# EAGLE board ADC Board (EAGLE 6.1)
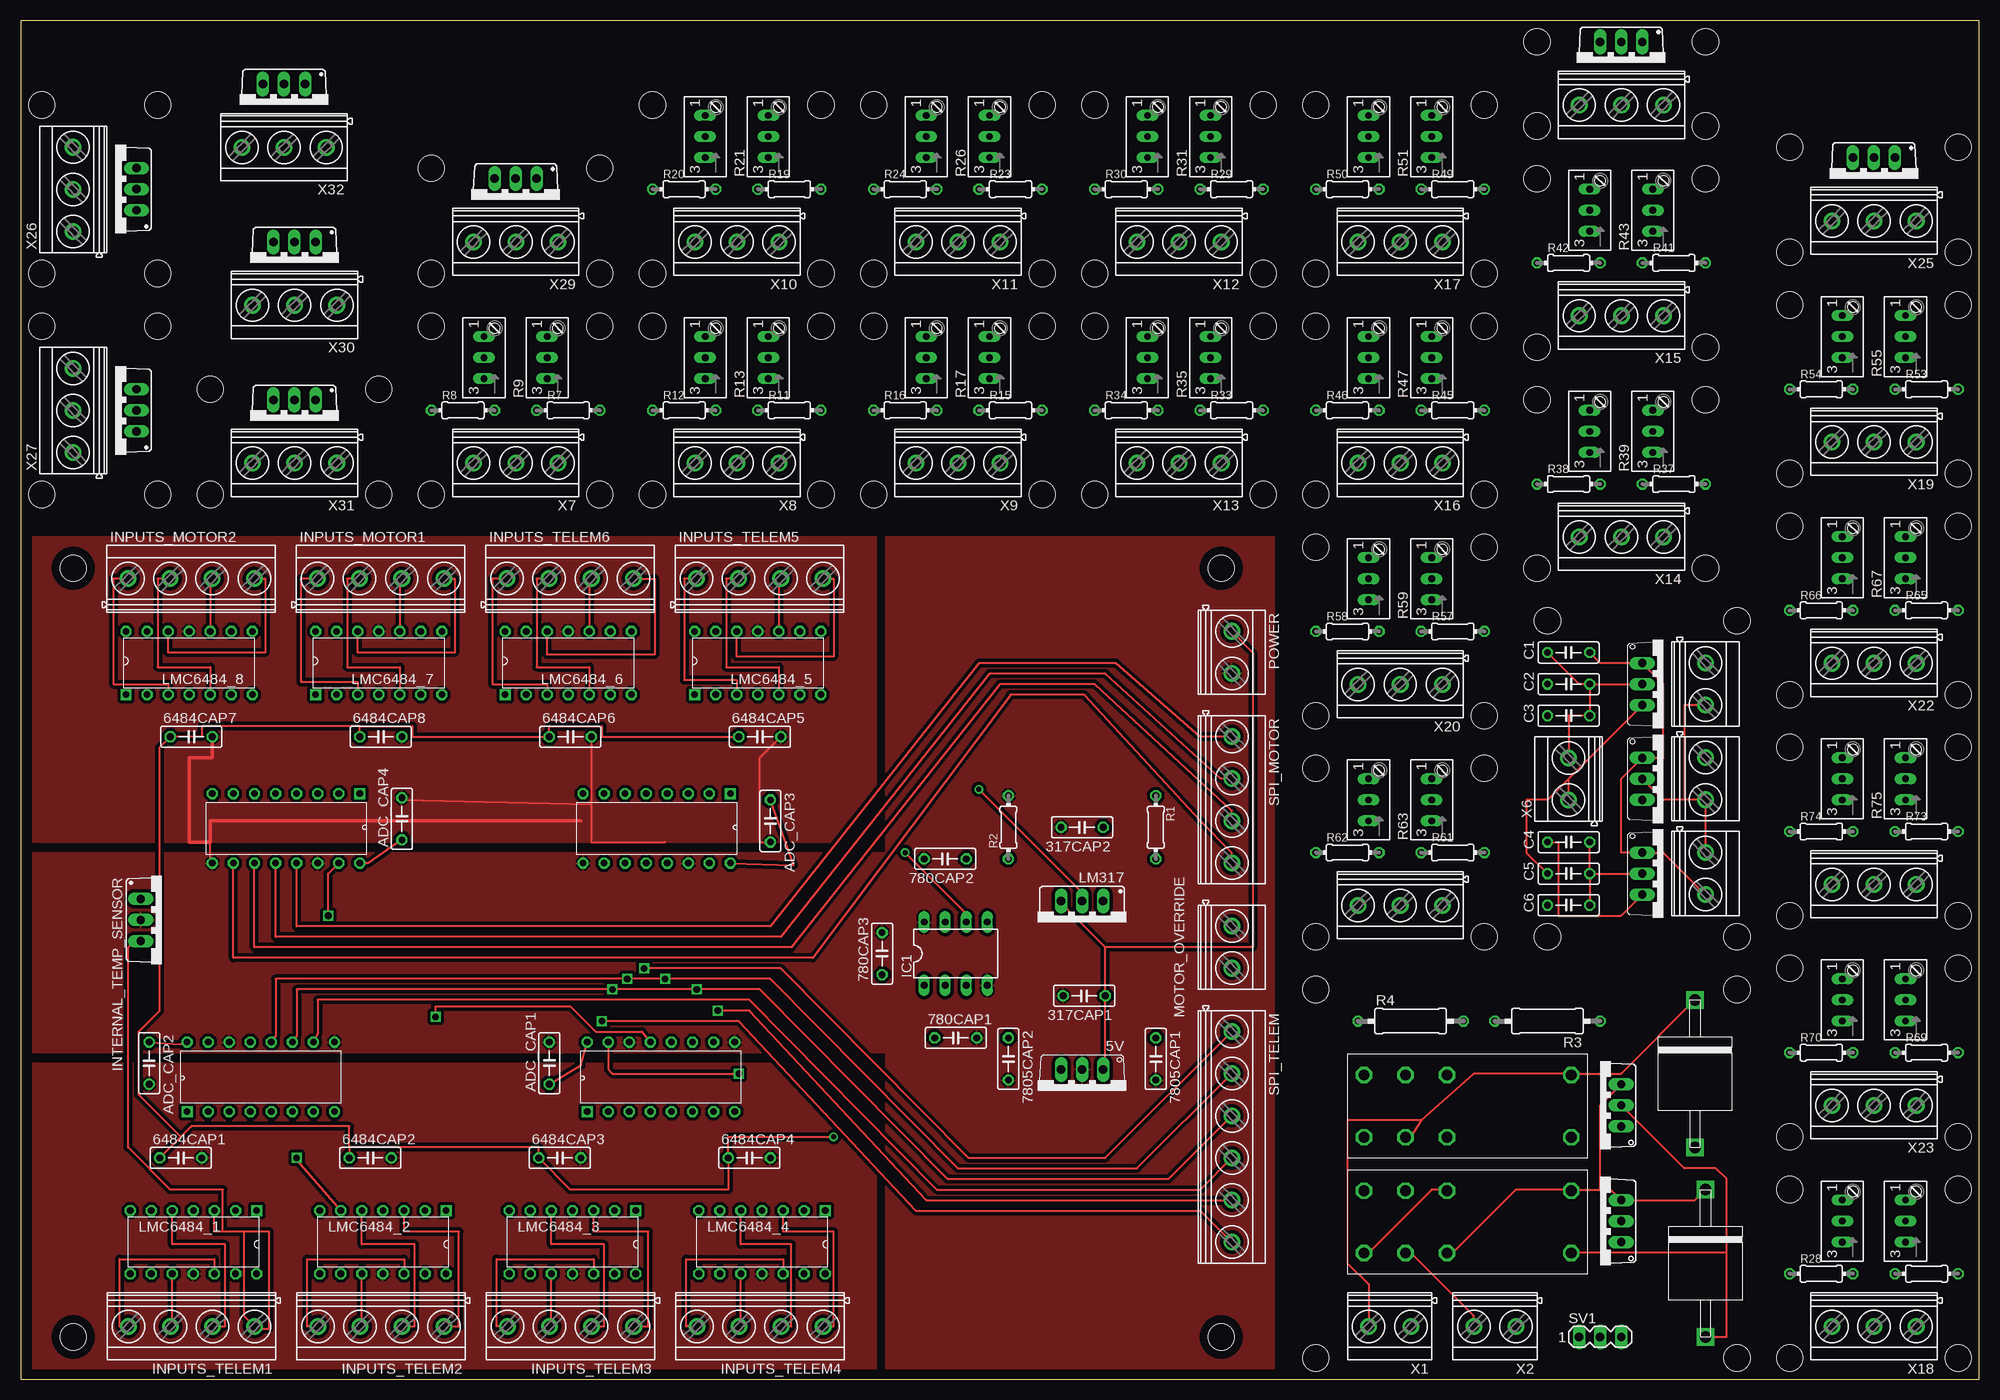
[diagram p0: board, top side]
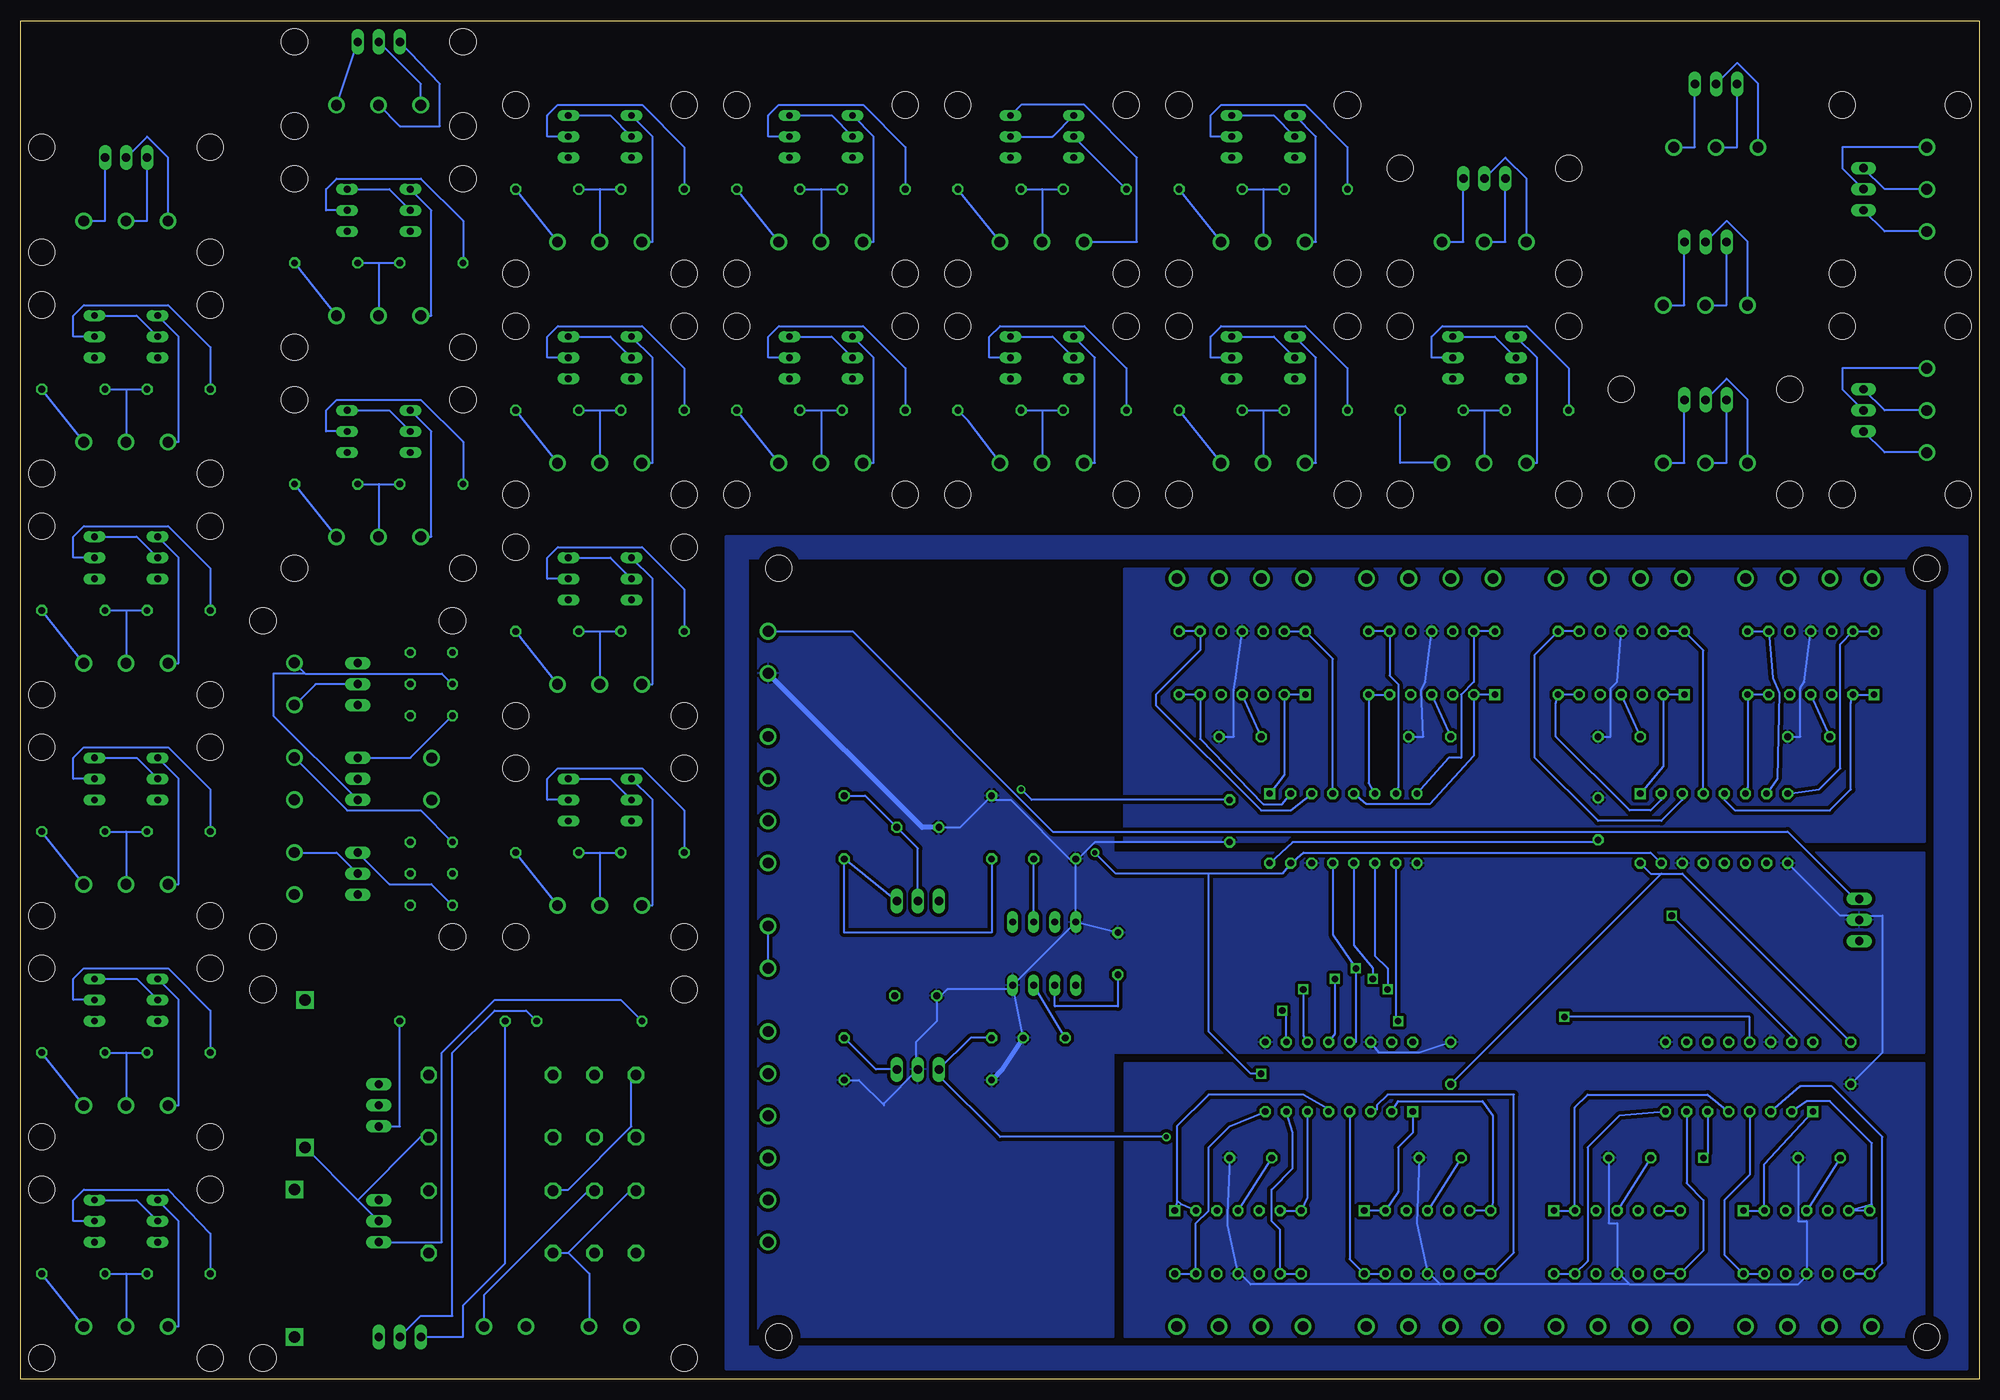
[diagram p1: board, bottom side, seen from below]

Size 236.23 x 163.83 mm. Coordinates in mm from the lower left corner, seen from the top.
Outline: 0,0 236.2,0 236.22,163.83 0,163.83 0,0
Copper layers (1*16): Top 0.035mm / dielectric 1.5mm / Bottom 0.035mm
Design rules: minimum track width 10mil, minimum drill 24mil, track to track 16mil, track to pad 8mil, pad to pad 8mil, via to via 8mil, smd to smd 8mil, copper to edge 40mil, drill to drill 8mil, minimum pad ring 10mil, minimum via ring 8mil, stop-mask expansion 4mil, vias tented up to drill 0mil, thermal gap 10mil
Holes 3.17 mm at 144.78,5.08 6.35,5.08 6.35,97.79 144.78,97.79 207.01,2.54 207.01,46.99 156.21,2.54 156.21,46.99 184.15,53.34 207.01,53.34 207.01,91.44 184.15,91.44 213.36,2.54 213.36,22.86 233.68,22.86 233.68,2.54 213.36,29.21 213.36,49.53 233.68,49.53 233.68,29.21 233.68,55.88 213.36,55.88 213.36,76.2 233.68,76.2 233.68,82.55 213.36,82.55 213.36,102.87 233.68,102.87 176.53,53.34 156.21,53.34 156.21,73.66 176.53,73.66 176.53,80.01 156.21,80.01 156.21,100.33 176.53,100.33 156.21,106.68 156.21,127 176.53,127 176.53,106.68 182.88,97.79 182.88,118.11 203.2,118.11 203.2,97.79 213.36,109.22 213.36,129.54 233.68,129.54 233.68,109.22 156.21,133.35 176.53,133.35 176.53,153.67 156.21,153.67 182.88,124.46 203.2,124.46 203.2,144.78 182.88,144.78 76.2,106.68 76.2,127 96.52,127 96.52,106.68 102.87,106.68 123.19,106.68 123.19,127 102.87,127 102.87,133.35 102.87,153.67 123.19,153.67 123.19,133.35 96.52,133.35 76.2,133.35 76.2,153.67 96.52,153.67 129.54,133.35 129.54,153.67 149.86,153.67 149.86,133.35 129.54,127 129.54,106.68 149.86,106.68 149.86,127 49.53,106.68 49.53,127 69.85,127 69.85,106.68 213.36,135.89 233.68,135.89 213.36,148.59 233.68,148.59 49.53,133.35 69.85,133.35 69.85,146.05 49.53,146.05 43.18,106.68 22.86,106.68 43.18,119.38 22.86,119.38 2.54,106.68 2.54,127 16.51,127 16.51,106.68 2.54,133.35 16.51,133.35 2.54,153.67 16.51,153.67 203.2,161.29 182.88,161.29 182.88,151.13 203.2,151.13

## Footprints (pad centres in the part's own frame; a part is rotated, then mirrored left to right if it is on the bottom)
TO220V = drill 1.016 long: 1 -2.54,-2.54; 2 0,-2.54; 3 2.54,-2.54
C050-025X075 = drill 0.813 octagon: 1 -2.54,0; 2 2.54,0
DIL08 = drill 0.813 long: 1 -3.81,-3.81; 2 -1.27,-3.81; 3 1.27,-3.81; 4 3.81,-3.81; 5 3.81,3.81; 6 1.27,3.81; 7 -1.27,3.81; 8 -3.81,3.81
MKDSN1,5/4-5,08 = drill 1.3 pad 2: 1 -7.641,0.025; 2 -2.561,0.025; 3 2.519,0.025; 4 7.599,0.025
TO220BV = drill 1.016 long: GND 0,-2.54; V+ -2.54,-2.54; VOUT 2.54,-2.54
317TS = drill 1.016 long: 1 -2.54,-2.54; 2 0,-2.54; 3 2.54,-2.54
JH924ABE = drill 0.813 square: 1 0,15.494 | drill 0.813 octagon: 2 0,12.954; 3 0,10.414; 4 0,7.874; 5 0,5.334; 6 0,2.794; 7 0,0.254; 8 7.62,0.254; 9 7.62,2.794; 10 7.62,5.334; 11 7.62,7.874; 12 7.62,10.414; 13 7.62,12.954; 14 7.62,15.494
MKDSN1,5/2-5,08 = drill 1.3 pad 2: 1 -2.561,0.025; 2 2.519,0.025
TO220AV = drill 1.016 long: B -2.54,-2.54; C 0,-2.54; E 2.54,-2.54
0204/7 = drill 0.813 octagon: 1 -3.81,0; 2 3.81,0
0309/12 = drill 0.813 octagon: 1 -6.35,0; 2 6.35,0
S64W = drill 0.813 long: A 2.54,1.27; E -2.54,1.27; S 0,1.27
MKDSN1,5/6-5,08 = drill 1.3 pad 2: 1 -12.7,0.025; 2 -7.62,0.025; 3 -2.54,0.025; 4 2.54,0.025; 5 7.62,0.025; 6 12.7,0.025
MA03-1 = drill 1.016 long: 1 -2.54,0; 2 0,0; 3 2.54,0
MCP3008 = drill 0.813 square: 1 -0.762,18.542 | drill 0.813 octagon: 2 -0.762,16.002; 3 -0.762,13.462; 4 -0.762,10.922; 5 -0.762,8.382; 6 -0.762,5.842; 7 -0.762,3.302; 8 -0.762,0.762; 9 7.62,0.762; 10 7.62,3.302; 11 7.62,5.842; 12 7.62,8.382; 13 7.62,10.922; 14 7.62,13.462; 15 7.62,16.002; 16 7.62,18.542
LM2-12D = drill 1.3 octagon: COIL1 27,2.5; COIL2 27,10; COM_1 7,2.5; COM_2 7,10; NC_1 12,10; NC_2 12,2.5; NO_1 2,10; NO_2 2,2.5
6A4 = drill 1.4 square: IN 0,0; OUT 17.78,0
MKDSN1,5/3-5,08 = drill 1.3 pad 2: 1 -7.641,0.025; 2 -2.561,0.025; 3 2.519,0.025

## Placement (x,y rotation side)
5V  LM7805TV  [TO220V]  128.02,34.8 180 top
317CAP1  .33uF  [C050-025X075]  128.27,46.23 180 top
317CAP2  1uF  [C050-025X075]  128.02,66.55 180 top
780CAP1  .1uF  [C050-025X075]  112.78,41.15 0 top
780CAP2  .1uF  [C050-025X075]  111.51,62.74 180 top
780CAP3  1uF  [C050-025X075]  103.89,51.31 90 top
6484CAP1  .1uF  [C050-025X075]  19.3,26.67 0 top
6484CAP2  .1uF  [C050-025X075]  42.16,26.67 0 top
6484CAP3  .1uF  [C050-025X075]  65.02,26.67 0 top
6484CAP4  .1uF  [C050-025X075]  87.88,26.67 0 top
6484CAP5  .1uF  [C050-025X075]  89.15,77.47 0 top
6484CAP6  .1uF  [C050-025X075]  66.29,77.47 0 top
6484CAP7  .1uF  [C050-025X075]  20.57,77.47 0 top
6484CAP8  .1uF  [C050-025X075]  43.43,77.47 0 top
7805CAP1  .33uF  [C050-025X075]  136.91,38.61 270 top
7805CAP2  1uF  [C050-025X075]  119.13,38.61 270 top
ADC_CAP1  .1uF  [C050-025X075]  63.75,38.1 90 top
ADC_CAP2  .1uF  [C050-025X075]  15.49,38.1 270 top
ADC_CAP3  .1uF  [C050-025X075]  90.42,67.31 270 top
ADC_CAP4  .1uF  [C050-025X075]  45.97,67.56 90 top
C1  [C050-025X075]  186.69,87.63 180 top
C2  [C050-025X075]  186.69,83.82 0 top
C3  [C050-025X075]  186.69,80.01 0 top
C4  [C050-025X075]  186.69,64.77 0 top
C5  [C050-025X075]  186.69,60.96 0 top
C6  [C050-025X075]  186.69,57.15 0 top
IC1  AD780N  [DIL08]  112.78,51.31 0 top
IC4  7805TV  [TO220V]  198.12,72.39 270 top
IC5  7805TV  [TO220V]  198.12,60.96 270 top
IC6  7805TV  [TO220V]  198.12,83.82 270 top
INPUTS_MOTOR1  [MKDSN1,5/4-5,08]  43.43,96.52 0 top
INPUTS_MOTOR2  [MKDSN1,5/4-5,08]  20.57,96.52 0 top
INPUTS_TELEM1  [MKDSN1,5/4-5,08]  20.57,6.35 180 top
INPUTS_TELEM2  [MKDSN1,5/4-5,08]  43.43,6.35 180 top
INPUTS_TELEM3  [MKDSN1,5/4-5,08]  66.29,6.35 180 top
INPUTS_TELEM4  [MKDSN1,5/4-5,08]  89.15,6.35 180 top
INPUTS_TELEM5  [MKDSN1,5/4-5,08]  89.15,96.52 0 top
INPUTS_TELEM6  [MKDSN1,5/4-5,08]  66.29,96.52 0 top
INTERNAL_TEMP_SENSOR  LM35  [TO220BV]  17.02,55.37 270 top
INTERNAL_TEMP_SENSOR1  LM35  [TO220BV]  223.52,144.78 180 top
INTERNAL_TEMP_SENSOR2  LM35  [TO220BV]  11.43,143.51 90 top
INTERNAL_TEMP_SENSOR3  LM35  [TO220BV]  11.43,116.84 90 top
INTERNAL_TEMP_SENSOR4  LM35  [TO220BV]  193.04,158.75 180 top
INTERNAL_TEMP_SENSOR5  LM35  [TO220BV]  59.69,142.24 180 top
INTERNAL_TEMP_SENSOR6  LM35  [TO220BV]  33.02,134.62 180 top
INTERNAL_TEMP_SENSOR7  LM35  [TO220BV]  33.02,115.57 180 top
INTERNAL_TEMP_SENSOR8  LM35  [TO220BV]  31.75,153.67 180 top
LM317  3.3v  [317TS]  128.02,55.12 180 top
LMC6484_1  JH924ABE  [JH924ABE]  12.95,20.32 270 top
LMC6484_2  JH924ABE  [JH924ABE]  35.81,20.32 270 top
LMC6484_3  JH924ABE  [JH924ABE]  58.67,20.32 270 top
LMC6484_4  JH924ABE  [JH924ABE]  81.53,20.32 270 top
LMC6484_5  JH924ABE  [JH924ABE]  96.77,82.55 90 top
LMC6484_6  JH924ABE  [JH924ABE]  73.91,82.55 90 top
LMC6484_7  JH924ABE  [JH924ABE]  51.05,82.55 90 top
LMC6484_8  JH924ABE  [JH924ABE]  28.19,82.55 90 top
MOTOR_OVERRIDE  [MKDSN1,5/2-5,08]  146.05,52.07 270 top
POWER  [MKDSN1,5/2-5,08]  146.05,87.63 270 top
Q1  MJE3055  [TO220AV]  190.5,33.02 90 top
Q2  MJE3055  [TO220AV]  190.5,19.05 90 top
R1  220  [0204/7]  136.91,66.55 270 top
R2  361  [0204/7]  119.13,66.55 90 top
R3  1K  [0309/12]  184.15,43.18 180 top
R4  1K  [0309/12]  167.64,43.18 0 top
R5  10K  [S64W]  228.6,19.05 90 top
R6  500  [S64W]  220.98,19.05 90 top
R7  1M  [0204/7]  66.04,116.84 0 top
R8  175K  [0204/7]  53.34,116.84 0 top
R9  50K  [S64W]  64.77,123.19 90 top
R10  2K  [S64W]  57.15,123.19 90 top
R11  1M  [0204/7]  92.71,116.84 0 top
R12  500K  [0204/7]  80.01,116.84 0 top
R13  200K  [S64W]  91.44,123.19 90 top
R14  10K  [S64W]  83.82,123.19 90 top
R15  1M  [0204/7]  119.38,116.84 0 top
R16  175K  [0204/7]  106.68,116.84 0 top
R17  50K  [S64W]  118.11,123.19 90 top
R18  2K  [S64W]  110.49,123.19 90 top
R19  1M  [0204/7]  92.71,143.51 0 top
R20  175K  [0204/7]  80.01,143.51 0 top
R21  50K  [S64W]  91.44,149.86 90 top
R22  2K  [S64W]  83.82,149.86 90 top
R23  1M  [0204/7]  119.38,143.51 0 top
R24  175K  [0204/7]  106.68,143.51 0 top
R25  50K  [S64W]  110.49,149.86 90 top
R26  2K  [S64W]  118.11,149.86 90 top
R27  1M  [0204/7]  229.87,12.7 0 top
R28  22K  [0204/7]  217.17,12.7 0 top
R29  1M  [0204/7]  146.05,143.51 0 top
R30  175K  [0204/7]  133.35,143.51 0 top
R31  50K  [S64W]  144.78,149.86 90 top
R32  2K  [S64W]  137.16,149.86 90 top
R33  1M  [0204/7]  146.05,116.84 0 top
R34  175K  [0204/7]  133.35,116.84 0 top
R35  50K  [S64W]  144.78,123.19 90 top
R36  2K  [S64W]  137.16,123.19 90 top
R37  1M  [0204/7]  199.39,107.95 0 top
R38  22K  [0204/7]  186.69,107.95 0 top
R39  10K  [S64W]  198.12,114.3 90 top
R40  500  [S64W]  190.5,114.3 90 top
R41  1M  [0204/7]  199.39,134.62 0 top
R42  22K  [0204/7]  186.69,134.62 0 top
R43  10K  [S64W]  198.12,140.97 90 top
R44  500  [S64W]  190.5,140.97 90 top
R45  1M  [0204/7]  172.72,116.84 0 top
R46  22K  [0204/7]  160.02,116.84 0 top
R47  10K  [S64W]  171.45,123.19 90 top
R48  500  [S64W]  163.83,123.19 90 top
R49  1M  [0204/7]  172.72,143.51 0 top
R50  22K  [0204/7]  160.02,143.51 0 top
R51  10K  [S64W]  171.45,149.86 90 top
R52  500  [S64W]  163.83,149.86 90 top
R53  1M  [0204/7]  229.87,119.38 0 top
R54  22K  [0204/7]  217.17,119.38 0 top
R55  10K  [S64W]  228.6,125.73 90 top
R56  500  [S64W]  220.98,125.73 90 top
R57  1M  [0204/7]  172.72,90.17 0 top
R58  500K  [0204/7]  160.02,90.17 0 top
R59  200K  [S64W]  171.45,96.52 90 top
R60  10K  [S64W]  163.83,96.52 90 top
R61  1M  [0204/7]  172.72,63.5 0 top
R62  500K  [0204/7]  160.02,63.5 0 top
R63  200K  [S64W]  171.45,69.85 90 top
R64  10K  [S64W]  163.83,69.85 90 top
R65  1M  [0204/7]  229.87,92.71 0 top
R66  500K  [0204/7]  217.17,92.71 0 top
R67  200K  [S64W]  228.6,99.06 90 top
R68  10K  [S64W]  220.98,99.06 90 top
R69  1M  [0204/7]  229.87,39.37 0 top
R70  500K  [0204/7]  217.17,39.37 0 top
R71  200K  [S64W]  228.6,45.72 90 top
R72  10K  [S64W]  220.98,45.72 90 top
R73  1M  [0204/7]  229.87,66.04 0 top
R74  500K  [0204/7]  217.17,66.04 0 top
R75  200K  [S64W]  228.6,72.39 90 top
R76  10K  [S64W]  220.98,72.39 90 top
SPI_MOTOR  [MKDSN1,5/4-5,08]  146.05,69.85 270 top
SPI_TELEM  [MKDSN1,5/6-5,08]  146.05,29.21 270 top
SV1  [MA03-1]  190.5,5.08 0 top
U$1  MCP3008  [MCP3008]  38.61,33.02 90 top
U$2  LM2-12D  [LM2-12D]  160.02,12.7 0 top
U$3  6A4  [6A4]  203.2,5.08 90 top
U$4  LM2-12D  [LM2-12D]  160.02,26.67 0 top
U$5  6A4  [6A4]  201.93,27.94 90 top
U$14  MCP3008  [MCP3008]  86.87,33.02 90 top
U$16  MCP3008  [MCP3008]  67.06,69.85 270 top
U$17  MCP3008  [MCP3008]  22.35,69.85 270 top
X1  MKDSN1,5/2-5,08  [MKDSN1,5/2-5,08]  165.1,6.35 180 top
X2  MKDSN1,5/2-5,08  [MKDSN1,5/2-5,08]  177.8,6.35 180 top
X3  MKDSN1,5/2-5,08  [MKDSN1,5/2-5,08]  203.2,60.96 270 top
X4  MKDSN1,5/2-5,08  [MKDSN1,5/2-5,08]  203.2,83.82 270 top
X5  MKDSN1,5/2-5,08  [MKDSN1,5/2-5,08]  203.2,72.39 270 top
X6  MKDSN1,5/2-5,08  [MKDSN1,5/2-5,08]  186.69,72.39 90 top
X7  MKDSN1,5/3-5,08  [MKDSN1,5/3-5,08]  57.15,110.49 180 top
X8  MKDSN1,5/3-5,08  [MKDSN1,5/3-5,08]  83.82,110.49 180 top
X9  MKDSN1,5/3-5,08  [MKDSN1,5/3-5,08]  110.49,110.49 180 top
X10  MKDSN1,5/3-5,08  [MKDSN1,5/3-5,08]  83.82,137.16 180 top
X11  MKDSN1,5/3-5,08  [MKDSN1,5/3-5,08]  110.49,137.16 180 top
X12  MKDSN1,5/3-5,08  [MKDSN1,5/3-5,08]  137.16,137.16 180 top
X13  MKDSN1,5/3-5,08  [MKDSN1,5/3-5,08]  137.16,110.49 180 top
X14  MKDSN1,5/3-5,08  [MKDSN1,5/3-5,08]  190.5,101.6 180 top
X15  MKDSN1,5/3-5,08  [MKDSN1,5/3-5,08]  190.5,128.27 180 top
X16  MKDSN1,5/3-5,08  [MKDSN1,5/3-5,08]  163.83,110.49 180 top
X17  MKDSN1,5/3-5,08  [MKDSN1,5/3-5,08]  163.83,137.16 180 top
X18  MKDSN1,5/3-5,08  [MKDSN1,5/3-5,08]  220.98,6.35 180 top
X19  MKDSN1,5/3-5,08  [MKDSN1,5/3-5,08]  220.98,113.03 180 top
X20  MKDSN1,5/3-5,08  [MKDSN1,5/3-5,08]  163.83,83.82 180 top
X21  MKDSN1,5/3-5,08  [MKDSN1,5/3-5,08]  163.83,57.15 180 top
X22  MKDSN1,5/3-5,08  [MKDSN1,5/3-5,08]  220.98,86.36 180 top
X23  MKDSN1,5/3-5,08  [MKDSN1,5/3-5,08]  220.98,33.02 180 top
X24  MKDSN1,5/3-5,08  [MKDSN1,5/3-5,08]  220.98,59.69 180 top
X25  MKDSN1,5/3-5,08  [MKDSN1,5/3-5,08]  220.98,139.7 180 top
X26  MKDSN1,5/3-5,08  [MKDSN1,5/3-5,08]  6.35,146.05 90 top
X27  MKDSN1,5/3-5,08  [MKDSN1,5/3-5,08]  6.35,119.38 90 top
X28  MKDSN1,5/3-5,08  [MKDSN1,5/3-5,08]  190.5,153.67 180 top
X29  MKDSN1,5/3-5,08  [MKDSN1,5/3-5,08]  57.15,137.16 180 top
X30  MKDSN1,5/3-5,08  [MKDSN1,5/3-5,08]  30.48,129.54 180 top
X31  MKDSN1,5/3-5,08  [MKDSN1,5/3-5,08]  30.48,110.49 180 top
X32  MKDSN1,5/3-5,08  [MKDSN1,5/3-5,08]  29.21,148.59 180 top

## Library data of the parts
5V IC4-IC6 = linear
317CAP1 317CAP2 780CAP1-780CAP3 6484CAP1-6484CAP8 7805CAP1 7805CAP2 ADC_CAP1-ADC_CAP4 C1-C6 R1-R4 R7 R8 R11 R12 R15 R16 R19 R20 R23 R24 R27-R30 R33 R34 R37 R38 R41 R42 R45 R46 R49 R50 R53 R54 R57 R58 R61 R62 R65 R66 R69 R70 R73 R74 = rcl
IC1 = analog-devices; MF: ALTERA CORPORATION; MPN: AD780ANZ; OC_FARNELL: 9605550; OC_NEWARK: 59K5478
INPUTS_MOTOR1 INPUTS_MOTOR2 INPUTS_TELEM1-INPUTS_TELEM6 SPI_MOTOR = con-phoenix-508; MPN: SMKDSN1,5/4-5,08; OC_FARNELL: 1792905; OC_NEWARK: 70R0300
INTERNAL_TEMP_SENSOR INTERNAL_TEMP_SENSOR1-INTERNAL_TEMP_SENSOR8 = ref-packages
LM317 = v-reg
LMC6484_1-LMC6484_8 = JH924
MOTOR_OVERRIDE POWER X1-X6 = con-phoenix-508; MPN: MKDSN 1,5/2-5.08; OC_FARNELL: 1792903; OC_NEWARK: 30M2397
Q1 Q2 = transistor-power
R5 R6 R9 R10 R13 R14 R17 R18 R21 R22 R25 R26 R31 R32 R35 R36 R39 R40 R43 R44 R47 R48 R51 R52 R55 R56 R59 R60 R63 R64 R67 R68 R71 R72 R75 R76 = pot
SPI_TELEM = con-phoenix-508; MPN: SMKDSN1,5/6-5,08; OC_FARNELL: 1792907; OC_NEWARK: 70R0302
SV1 = con-lstb; OC_FARNELL: unknown; OC_NEWARK: unknown
U$1 U$14 U$16 U$17 = mcp300X
U$2-U$5 = SolarJackets
X7-X32 = con-phoenix-508; MPN: SMKDSN1,5/3-5,08; OC_FARNELL: 1792904; OC_NEWARK: 70R0299

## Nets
3.3V: 317CAP2.1 ADC_CAP1.1 ADC_CAP2.1 ADC_CAP3.1 ADC_CAP4.1 LM317.2 R1.1 U$1.16 U$14.16 U$16.16 U$17.16
5V: 5V.3 6484CAP1.1 6484CAP2.1 6484CAP3.1 6484CAP4.1 6484CAP5.1 6484CAP6.1 6484CAP7.1 6484CAP8.1 7805CAP2.1 LMC6484_1.4 LMC6484_2.4 LMC6484_3.4 LMC6484_4.4 LMC6484_5.4 LMC6484_6.4 LMC6484_7.4 LMC6484_8.4
12V: 5V.1 317CAP1.1 7805CAP1.1 INTERNAL_TEMP_SENSOR.V+ LM317.3 POWER.1
12V1: U$4.COIL2 U$4.COM_1 U$5.OUT X1.2
+5V: 780CAP3.1 IC1.2
A0: LMC6484_1.1 LMC6484_1.2 U$1.1
A1: LMC6484_1.6 LMC6484_1.7 U$1.2
A2: LMC6484_1.8 LMC6484_1.9 U$1.3
A3: LMC6484_1.13 LMC6484_1.14 U$1.4
A4: LMC6484_2.1 LMC6484_2.2 U$1.5
A5: LMC6484_2.6 LMC6484_2.7 U$1.6
A6: LMC6484_2.8 LMC6484_2.9 U$1.7
A7: LMC6484_2.13 LMC6484_2.14 U$1.8
A8: LMC6484_3.1 LMC6484_3.2 U$14.1
A9: LMC6484_3.6 LMC6484_3.7 U$14.2
A10: LMC6484_3.8 LMC6484_3.9 U$14.3
A11: LMC6484_3.13 LMC6484_3.14 U$14.4
A12: LMC6484_4.1 LMC6484_4.2 U$14.5
A13: LMC6484_4.6 LMC6484_4.7 U$14.6
A14: LMC6484_4.8 LMC6484_4.9 U$14.7
A15: LMC6484_4.13 LMC6484_4.14 U$14.8
A16: LMC6484_5.1 LMC6484_5.2 U$16.1
A17: LMC6484_5.6 LMC6484_5.7 U$16.2
A18: LMC6484_5.8 LMC6484_5.9 U$16.3
A19: LMC6484_5.13 LMC6484_5.14 U$16.4
A20: LMC6484_6.1 LMC6484_6.2 U$16.5
A21: LMC6484_6.6 LMC6484_6.7 U$16.6
A22: LMC6484_6.8 LMC6484_6.9 U$16.7
A23: LMC6484_6.13 LMC6484_6.14 U$16.8
A24: LMC6484_7.1 LMC6484_7.2 U$17.1
A25: LMC6484_7.6 LMC6484_7.7 U$17.2
A26: LMC6484_7.8 LMC6484_7.9 U$17.3
A27: LMC6484_7.13 LMC6484_7.14 U$17.4
A28: LMC6484_8.1 LMC6484_8.2 U$17.5
A29: LMC6484_8.6 LMC6484_8.7 U$17.6
A30: LMC6484_8.8 LMC6484_8.9 U$17.7
A31: LMC6484_8.13 LMC6484_8.14 U$17.8
GND: 5V.2 317CAP1.2 317CAP2.2 780CAP1.2 780CAP2.2 780CAP3.2 6484CAP1.2 6484CAP2.2 6484CAP3.2 6484CAP4.2 6484CAP5.2 6484CAP6.2 6484CAP7.2 6484CAP8.2 7805CAP1.2 7805CAP2.2 ADC_CAP1.2 ADC_CAP2.2 ADC_CAP3.2 ADC_CAP4.2 IC1.4 IC1.8 INTERNAL_TEMP_SENSOR.GND LMC6484_1.11 LMC6484_2.11 LMC6484_3.11 LMC6484_4.11 LMC6484_5.11 LMC6484_6.11 LMC6484_7.11 LMC6484_8.11 POWER.2 R2.2 U$1.9 U$1.14 U$14.9 U$14.14 U$16.9 U$16.14 U$17.9 U$17.14
GND1: Q1.E Q2.E U$2.COIL2 U$2.NC_2 U$2.NO_1 U$3.OUT X1.1
GREEN: U$2.COM_2 X2.1
IN1: INPUTS_TELEM1.1 INTERNAL_TEMP_SENSOR.VOUT LMC6484_1.3
IN2: INPUTS_TELEM1.2 LMC6484_1.5
IN3: INPUTS_TELEM1.3 LMC6484_1.10
IN4: INPUTS_TELEM1.4 LMC6484_1.12
IN5: INPUTS_TELEM2.1 LMC6484_2.3
IN6: INPUTS_TELEM2.2 LMC6484_2.5
IN7: INPUTS_TELEM2.3 LMC6484_2.10
IN8: INPUTS_TELEM2.4 LMC6484_2.12
IN9: INPUTS_TELEM3.1 LMC6484_3.3
IN10: INPUTS_TELEM3.2 LMC6484_3.5
IN11: INPUTS_TELEM3.3 LMC6484_3.10
IN13: INPUTS_TELEM4.1 LMC6484_4.3
IN14: INPUTS_TELEM4.2 LMC6484_4.5
IN15: INPUTS_TELEM4.3 LMC6484_4.10
IN16: INPUTS_TELEM4.4 LMC6484_4.12
IN17: INPUTS_TELEM5.1 LMC6484_5.3
IN18: INPUTS_TELEM5.2 LMC6484_5.5
IN19: INPUTS_TELEM5.3 LMC6484_5.10
IN20: INPUTS_TELEM5.4 LMC6484_5.12
IN21: INPUTS_TELEM6.1 LMC6484_6.3
IN22: INPUTS_TELEM6.2 LMC6484_6.5
IN23: INPUTS_TELEM6.3 LMC6484_6.10
IN24: INPUTS_TELEM6.4 LMC6484_6.12
IN25: INPUTS_MOTOR1.1 LMC6484_7.3
IN26: INPUTS_MOTOR1.2 LMC6484_7.5
IN27: INPUTS_MOTOR1.3 LMC6484_7.10
IN28: INPUTS_MOTOR1.4 LMC6484_7.12
IN29: INPUTS_MOTOR2.1 LMC6484_8.3
IN30: INPUTS_MOTOR2.2 LMC6484_8.5
IN31: INPUTS_MOTOR2.3 LMC6484_8.10
IN32: INPUTS_MOTOR2.4 LMC6484_8.12
MOTOR_OVERRIDE: MOTOR_OVERRIDE.1 MOTOR_OVERRIDE.2
N$1: LM317.1 R1.2 R2.1
N$2: U$2.NC_1 U$2.NO_2 U$4.NO_1
N$3: 780CAP1.1 IC1.3
N$4: Q1.C U$2.COIL1 U$3.IN
N$5: R4.2 SV1.2
N$6: Q2.C U$4.COIL1 U$5.IN
N$7: Q1.B R3.1
N$8: R3.2 SV1.1
N$9: Q2.B R4.1
N$10: C1.2 C2.2 C3.2 C4.2 C5.2 C6.2 IC4.2 IC5.2 IC6.2 X3.1 X4.2 X5.2 X6.2
N$11: C2.1 IC4.3 X4.1
N$12: C4.1 IC5.3 X5.1
N$13: C5.1 IC6.3 X6.1
N$14: INPUTS_TELEM3.4 LMC6484_3.12
N$15: C1.1 C3.1 C6.1 IC4.1 IC5.1 IC6.1 X3.2
N$16: R5.A R6.S
N$17: R6.A X18.3
N$18: R27.2 X18.1
N$19: R5.S R28.1
N$20: R7.1 R8.2 X7.2
N$21: R8.1 R9.S
N$22: R9.A R10.S
N$23: R10.A X7.3
N$24: R7.2 X7.1
N$25: R11.1 R12.2 X8.2
N$26: R12.1 R13.S
N$27: R13.A R14.S
N$28: R14.A X8.3
N$29: R11.2 X8.1
N$30: R15.1 R16.2 X9.2
N$31: R16.1 R17.S
N$32: R17.A R18.S
N$33: R18.A X9.3
N$34: R15.2 X9.1
N$35: R19.1 R20.2 X10.2
N$36: R20.1 R21.S
N$37: R21.A R22.S
N$38: R22.A X10.3
N$39: R19.2 X10.1
N$40: R23.1 R24.2 X11.2
N$41: R24.1 R25.S
N$42: R25.A R26.S
N$43: R26.A X11.3
N$44: R23.2 X11.1
N$45: R29.1 R30.2 X12.2
N$46: R30.1 R31.S
N$47: R31.A R32.S
N$48: R32.A X12.3
N$49: R27.1 R28.2 X18.2
N$50: R29.2 X12.1
N$51: R33.1 R34.2 X13.2
N$52: R34.1 R35.S
N$53: R35.A R36.S
N$54: R36.A X13.3
N$55: R33.2 X13.1
N$56: R37.1 R38.2 X14.2
N$57: R38.1 R39.S
N$58: R39.A R40.S
N$59: R40.A X14.3
N$60: R37.2 X14.1
N$61: R41.1 R42.2 X15.2
N$62: R42.1 R43.S
N$63: R43.A R44.S
N$64: R44.A X15.3
N$65: R41.2 X15.1
N$66: R45.1 R46.2 X16.2
N$67: R46.1 R47.S
N$68: R47.A R48.S
N$69: R48.A X16.3
N$70: R45.2 X16.1
N$71: R49.1 R50.2 X17.2
N$72: R50.1 R51.S
N$73: R51.A R52.S
N$74: R52.A X17.3
N$75: R49.2 X17.1
N$76: R53.1 R54.2 X19.2
N$77: R54.1 R55.S
N$78: R55.A R56.S
N$79: R56.A X19.3
N$80: R53.2 X19.1
N$81: R57.1 R58.2 X20.2
N$82: R58.1 R59.S
N$83: R59.A R60.S
N$84: R60.A X20.3
N$85: R57.2 X20.1
N$86: R61.1 R62.2 X21.2
N$87: R62.1 R63.S
N$88: R63.A R64.S
N$89: R64.A X21.3
N$90: R61.2 X21.1
N$91: R65.1 R66.2 X22.2
N$92: R66.1 R67.S
N$93: R67.A R68.S
N$94: R68.A X22.3
N$95: R65.2 X22.1
N$96: R69.1 R70.2 X23.2
N$97: R70.1 R71.S
N$98: R71.A R72.S
N$99: R72.A X23.3
N$100: R69.2 X23.1
N$101: R73.1 R74.2 X24.2
N$102: R74.1 R75.S
N$103: R75.A R76.S
N$104: R76.A X24.3
N$105: R73.2 X24.1
N$106: INTERNAL_TEMP_SENSOR1.V+ X25.1
N$107: INTERNAL_TEMP_SENSOR1.VOUT X25.2
N$108: INTERNAL_TEMP_SENSOR1.GND X25.3
N$109: INTERNAL_TEMP_SENSOR2.V+ X26.1
N$110: INTERNAL_TEMP_SENSOR2.VOUT X26.2
N$111: INTERNAL_TEMP_SENSOR2.GND X26.3
N$112: INTERNAL_TEMP_SENSOR3.V+ X27.1
N$113: INTERNAL_TEMP_SENSOR3.VOUT X27.2
N$114: INTERNAL_TEMP_SENSOR3.GND X27.3
N$115: INTERNAL_TEMP_SENSOR4.V+ X28.1
N$116: INTERNAL_TEMP_SENSOR4.VOUT X28.2
N$117: INTERNAL_TEMP_SENSOR4.GND X28.3
N$118: INTERNAL_TEMP_SENSOR5.V+ X29.1
N$119: INTERNAL_TEMP_SENSOR5.VOUT X29.2
N$120: INTERNAL_TEMP_SENSOR5.GND X29.3
N$121: INTERNAL_TEMP_SENSOR6.V+ X30.1
N$122: INTERNAL_TEMP_SENSOR6.VOUT X30.2
N$123: INTERNAL_TEMP_SENSOR6.GND X30.3
N$124: INTERNAL_TEMP_SENSOR7.V+ X31.1
N$125: INTERNAL_TEMP_SENSOR7.VOUT X31.2
N$126: INTERNAL_TEMP_SENSOR7.GND X31.3
N$127: INTERNAL_TEMP_SENSOR8.V+ X32.1
N$128: INTERNAL_TEMP_SENSOR8.VOUT X32.2
N$129: INTERNAL_TEMP_SENSOR8.GND X32.3
PURPLE: U$2.COM_1 X2.2
SPI_CLK: SPI_TELEM.1 U$1.13 U$14.13 U$16.13
SPI_CLK_MOTOR: SPI_MOTOR.1 U$17.13
SPI_CS1: SPI_TELEM.4 U$1.10
SPI_CS2: SPI_TELEM.5 U$14.10
SPI_CS3: SPI_TELEM.6 U$16.10
SPI_CS4: SPI_MOTOR.4 U$17.10
SPI_DIN: SPI_TELEM.3 U$1.11 U$14.11 U$16.11
SPI_DIN_MOTOR: SPI_MOTOR.3 U$17.11
SPI_DOUT: SPI_TELEM.2 U$1.12 U$14.12 U$16.12
SPI_DOUT_MOTOR: SPI_MOTOR.2 U$17.12
VREF: 780CAP2.1 IC1.6 U$1.15 U$14.15 U$16.15 U$17.15

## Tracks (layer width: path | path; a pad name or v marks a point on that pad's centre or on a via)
3.3V  (via drill 0.61)
  Top 0.254: U$16.16 93.22,61.98 ADC_CAP3.1 | ADC_CAP1.1 67.56,37.85 U$14.16 | ADC_CAP4.1 41.91,62.23 U$17.16 | ADC_CAP2.1 19.3,40.39 U$1.16 | v115.57,71.12 128.27,58.42 LM317.2
  Bottom 0.254: R1.1 134.37,70.36 317CAP2.1 128.02,64.01 LM317.2 | ADC_CAP2.1 35.81,60.96 38.35,60.96 | 38.35,60.96 39.62,60.96 U$17.16 | 38.35,60.96 ADC_CAP1.1 | U$16.16 82.8,64.77 45.97,64.77 ADC_CAP4.1 | v115.57,71.12 114.3,69.85 ADC_CAP3.1
5V  (via drill 0.61)
  Top 0.254: 40.89,78.74 21.84,78.74 21.84,77.47 6484CAP7.1 16.76,76.2 16.76,44.45 14.22,41.91 14.22,34.29 19.3,29.21 | 6484CAP8.1 40.89,78.74 | 40.89,78.74 47.24,78.74 47.24,77.47 6484CAP6.1 63.75,78.74 70.1,78.74 70.1,77.47 6484CAP5.1 | 19.3,29.21 20.57,30.48 39.62,30.48 39.62,27.94 | 19.3,29.21 6484CAP1.1 | v98.04,29.21 85.34,29.21 6484CAP4.1 85.34,22.86 66.29,22.86 6484CAP3.1 62.48,27.94 39.62,27.94 | 39.62,27.94 6484CAP2.1
  Bottom 0.254: 6484CAP5.1 LMC6484_5.4 | LMC6484_8.4 6484CAP7.1 | LMC6484_7.4 6484CAP8.1 | LMC6484_6.4 6484CAP6.1 | 6484CAP1.1 LMC6484_1.4 | 6484CAP2.1 LMC6484_2.4 | 6484CAP3.1 LMC6484_3.4 | 6484CAP4.1 LMC6484_4.4 | 7805CAP2.1 121.67,41.15 5V.3 125.73,36.83 118.11,29.21 v98.04,29.21
12V
  Top 0.254: 5V.1 130.81,38.1 317CAP1.1 130.81,52.07 | 130.81,52.07 125.73,57.15 LM317.3 | 130.81,52.07 148.59,52.07 148.59,87.63 146.05,90.17 POWER.1
  Bottom 0.254: 5V.1 133.1,37.34 7805CAP1.1 | INTERNAL_TEMP_SENSOR.V+ 15.49,58.42 23.11,66.04 111.76,66.04 135.89,90.17 146.05,90.17 POWER.1
12V1
  Top 0.254: 168.91,31.24 175.26,36.83 186.69,36.83 U$4.COIL2 187.96,36.83 193.04,36.83 U$5.OUT | 168.91,31.24 167.64,29.21 U$4.COM_1 | 168.91,31.24 160.02,31.24 160.02,13.97 162.56,11.43 162.56,6.35 X1.2
+5V
  Bottom 0.254: 780CAP3.1 103.89,44.96 111.51,44.96 IC1.2
A0
  Bottom 0.254: LMC6484_1.1 LMC6484_1.2 25.91,25.91 U$1.1
A1
  Bottom 0.254: LMC6484_1.7 LMC6484_1.6 12.95,21.08 12.95,28.45 18.03,33.53 20.83,33.53 U$1.2
A2
  Bottom 0.254: LMC6484_1.8 LMC6484_1.9 12.95,12.7 11.68,13.97 11.68,29.21 17.78,35.31 21.59,35.31 U$1.3
A3
  Bottom 0.254: U$1.4 27.69,24.64 30.73,21.59 30.73,14.99 LMC6484_1.14 LMC6484_1.13
A4
  Bottom 0.254: LMC6484_2.1 LMC6484_2.2 48.77,32.77 47.24,34.29 32.77,34.29 U$1.5
A5  (via drill 0.8)
  Top 0.254: v33.27,26.67 33.27,26.42 LMC6484_2.6
  Bottom 0.254: LMC6484_2.6 LMC6484_2.7 | U$1.6 32.77,27.18 v33.27,26.67
A6
  Bottom 0.254: U$1.7 35.31,23.62 33.27,21.59 33.27,15.49 LMC6484_2.8 LMC6484_2.9
A7
  Bottom 0.254: LMC6484_2.14 LMC6484_2.13 47.24,14.22 47.24,27.94 43.43,31.75 U$1.8
A8
  Bottom 0.254: U$14.1 68.33,29.72 70.1,27.94 70.1,22.61 LMC6484_3.2 LMC6484_3.1
A9
  Bottom 0.254: U$14.2 70.1,33.53 59.94,33.53 58.67,31.75 58.67,21.34 LMC6484_3.7 LMC6484_3.6
A10
  Bottom 0.254: LMC6484_3.8 LMC6484_3.9 58.67,12.7 56.13,15.24 56.13,34.29 71.37,34.29 72.64,33.02 72.64,32.51 U$14.3
A11
  Bottom 0.254: U$14.4 75.95,14.48 LMC6484_3.14 LMC6484_3.13
A12
  Bottom 0.254: U$14.5 78.49,32.51 81.53,34.29 92.96,34.29 96.77,30.48 96.77,21.59 | 96.77,21.59 96.77,21.34 LMC6484_4.1 | LMC6484_4.2 96.27,21.08 96.77,21.59
A13
  Bottom 0.254: U$14.6 81.03,21.84 LMC6484_4.7 LMC6484_4.6
A14
  Bottom 0.254: LMC6484_4.8 LMC6484_4.9 84.33,18.03 85.34,19.05 85.34,22.86 82.8,25.4 82.8,29.72 U$14.7
A15
  Bottom 0.254: LMC6484_4.14 LMC6484_4.13 94.49,18.8 92.96,20.32 92.96,27.94 90.42,30.48 U$14.8
A16
  Bottom 0.254: LMC6484_5.1 LMC6484_5.2 83.82,72.9 U$16.1
A17
  Bottom 0.254: LMC6484_5.7 LMC6484_5.6 93.98,77.22 86.36,69.34 84.07,69.34 U$16.2
A18
  Bottom 0.254: LMC6484_5.8 LMC6484_5.9 93.98,87.88 99.31,82.55 99.31,81.28 86.61,68.58 83.06,68.58 U$16.3
A19
  Bottom 0.254: U$16.4 77.98,86.87 LMC6484_5.14 LMC6484_5.13 84.07,90.17
A20
  Bottom 0.254: LMC6484_6.1 LMC6484_6.2 60.96,75.18 66.29,69.34 73.91,69.34 U$16.5
A21
  Bottom 0.254: LMC6484_6.6 LMC6484_6.7 73.66,71.88 U$16.6
A22
  Bottom 0.254: LMC6484_6.8 LMC6484_6.9 71.12,84.84 70.1,83.82 70.1,71.37 U$16.7
A23
  Bottom 0.254: LMC6484_6.14 LMC6484_6.13 60.96,84.07 62.48,82.55 62.48,74.93 64.01,74.93 U$16.8
A24
  Bottom 0.254: LMC6484_7.1 LMC6484_7.2 38.1,73.91 U$17.1
A25
  Bottom 0.254: LMC6484_7.6 LMC6484_7.7 51.05,81.53 51.05,77.47 42.16,68.58 39.62,68.58 38.35,69.85 U$17.2
A26
  Bottom 0.254: LMC6484_7.9 LMC6484_7.8 53.59,87.38 53.59,74.93 45.97,67.31 38.35,67.31 35.81,69.85 U$17.3
A27
  Bottom 0.254: LMC6484_7.13 LMC6484_7.14 33.27,87.88 U$17.4
A28
  Bottom 0.254: LMC6484_8.1 LMC6484_8.2 15.49,81.53 15.49,71.12 18.03,68.58 29.46,68.58 30.73,69.85 U$17.5
A29
  Bottom 0.254: LMC6484_8.6 LMC6484_8.7 27.94,71.37 U$17.6
A30
  Bottom 0.254: LMC6484_8.8 LMC6484_8.9 24.89,84.58 24.13,82.8 24.38,72.39 U$17.7
A31
  Bottom 0.254: U$17.8 19.3,71.12 16.76,73.66 16.76,88.65 LMC6484_8.13 LMC6484_8.14
GND
  Top 0.254: ADC_CAP3.2 89.16,64.74 89.15,64.77 89.15,74.93 6484CAP5.2 | 6484CAP6.2 68.83,69.34 | 68.83,69.34 68.83,64.77 77.72,64.77 | 67.56,62.23 U$16.9 | 68.83,69.34 45.97,69.85 ADC_CAP4.2 | U$17.9 22.86,62.23 22.86,64.77
  Top 0.406: 67.56,67.31 22.86,67.31 22.86,64.77 20.32,64.77 20.32,74.93 23.11,74.93 6484CAP7.2
  Bottom 0.254: 6484CAP7.2 21.59,77.47 21.59,83.31 21.08,84.07 LMC6484_8.11 | 6484CAP8.2 44.45,77.47 44.45,83.31 43.69,84.07 LMC6484_7.11 | 6484CAP5.2 89.92,77.47 89.92,83.06 89.66,84.58 LMC6484_5.11 | 6484CAP6.2 67.06,77.47 67.31,83.06 66.8,84.07 LMC6484_6.11 | 6484CAP1.2 21.84,19.05 20.83,19.05 LMC6484_1.11 20.57,12.7 21.84,11.43 42.16,11.43 | 6484CAP2.2 44.7,18.8 43.69,18.8 LMC6484_2.11 43.43,12.7 42.16,11.43 | 6484CAP3.2 67.82,18.8 LMC6484_3.11 66.29,12.7 65.02,11.43 | 6484CAP4.2 90.68,19.81 90.68,18.54 LMC6484_4.11 89.15,12.7 87.88,11.43 65.02,11.43 | IC1.8 780CAP2.2 109.22,62.23 | 780CAP3.2 IC1.8 | IC1.4 IC1.8 | 780CAP1.2 IC1.4 | 317CAP2.2 122.94,66.55 R2.2 119.38,69.85 116.84,69.85 109.22,62.23 | 125.73,45.72 125.73,43.18 128.27,40.64 128.27,37.59 5V.2 132.08,33.27 132.08,33.02 135.13,36.07 7805CAP1.2 | ADC_CAP1.2 67.56,39.37 72.39,39.37 U$14.14 | 125.73,45.72 124.46,46.99 116.84,46.99 IC1.4 | 125.73,45.72 317CAP1.2 | 146.05,85.09 POWER.2 | 42.16,11.43 65.02,11.43 | U$17.9 16.76,55.88 15.49,55.88 INTERNAL_TEMP_SENSOR.GND 14.22,55.88 11.68,55.88 11.68,39.37 ADC_CAP2.2 | 109.22,62.23 106.68,64.77 ADC_CAP3.2
  Bottom 0.61: 780CAP1.2 117.86,37.34 7805CAP2.2 | 317CAP2.2 127.51,66.55 146.05,85.09
  pour Bottom: 6.6,63.5 104.39,63.5 104.39,97.79 147.32,97.79 147.32,5.08 104.39,5.08 104.39,39.37 6.6,39.37
  pour Bottom: 6.6,38.1 103.12,38.1 103.12,5.08 6.6,5.08
  pour Bottom: 6.6,97.79 6.6,64.77 103.12,64.77 103.12,97.79
  pour Top: 1.52,101.6 103.12,101.6 103.12,64.77 1.52,64.77
  pour Top: 1.52,1.27 1.52,38.1 103.12,38.1 103.12,1.27
  pour Top: 1.52,63.5 104.39,63.5 104.39,101.6 151.13,101.6 151.13,1.27 104.39,1.27 104.39,39.37 1.52,39.37
GND1
  Top 0.254: 190.5,22.86 187.96,22.86 U$2.COIL2 186.69,22.86 180.34,22.86 172.72,15.24 U$2.NC_2 | 190.5,22.86 191.77,22.86 Q2.E 201.93,21.59 U$3.OUT | Q1.E 190.5,33.02 190.5,22.86
  Bottom 0.254: 170.18,15.24 162.56,22.86 U$2.NO_1 | 170.18,15.24 171.45,15.24 U$2.NC_2 | 170.18,15.24 167.64,12.7 167.64,6.35 X1.1
GREEN
  Bottom 0.254: U$2.COM_2 167.64,22.86 180.34,10.16 180.34,6.35 X2.1
IN1
  Top 0.254: 28.19,6.1 29.97,6.1 29.97,17.78 26.92,17.78 | 26.92,17.78 24.38,17.78 | 24.38,17.78 23.37,17.78 LMC6484_1.3 | 24.38,17.78 24.38,22.86 18.03,22.86 12.95,27.94 12.95,52.07 14.22,53.34 INTERNAL_TEMP_SENSOR.VOUT | 26.92,17.78 26.92,7.62 28.19,6.35 INPUTS_TELEM1.1
IN2
  Top 0.254: LMC6484_1.5 18.29,16.26 24.64,16.26 24.64,6.35 23.11,6.35 INPUTS_TELEM1.2
IN3
  Top 0.254: LMC6484_1.10 18.29,6.35 18.03,6.35 INPUTS_TELEM1.3
IN4
  Top 0.254: LMC6484_1.12 23.37,14.48 11.94,14.48 11.94,6.35 12.95,6.35 INPUTS_TELEM1.4
IN5
  Top 0.254: LMC6484_2.3 46.23,17.78 52.83,17.78 52.83,6.35 51.05,6.35 INPUTS_TELEM2.1
IN6
  Top 0.254: LMC6484_2.5 41.15,16.26 47.5,16.26 47.5,6.35 45.97,6.35 INPUTS_TELEM2.2
IN7
  Top 0.254: LMC6484_2.10 41.15,6.35 40.89,6.35 INPUTS_TELEM2.3
IN8
  Top 0.254: 36.07,6.35 35.81,6.35 | 35.81,6.35 34.54,6.35 34.54,14.48 46.23,14.48 LMC6484_2.12 | 35.81,6.35 INPUTS_TELEM2.4
IN9
  Top 0.254: LMC6484_3.3 69.09,17.78 75.69,17.78 75.69,6.35 73.91,6.35 INPUTS_TELEM3.1
IN10
  Top 0.254: LMC6484_3.5 64.01,16.26 70.36,16.26 70.36,6.35 68.83,6.35 INPUTS_TELEM3.2
IN11
  Top 0.254: LMC6484_3.10 64.01,6.35 63.75,6.35 INPUTS_TELEM3.3
IN13
  Top 0.254: LMC6484_4.3 91.95,17.78 98.04,17.78 98.04,6.35 96.77,6.35 INPUTS_TELEM4.1
IN14
  Top 0.254: LMC6484_4.5 86.87,16.26 92.96,16.26 92.96,6.35 91.69,6.35 INPUTS_TELEM4.2
IN15
  Top 0.254: LMC6484_4.10 86.87,6.35 86.61,6.35 INPUTS_TELEM4.3
IN16
  Top 0.254: LMC6484_4.12 91.95,14.48 80.26,14.48 80.26,6.35 81.53,6.35 INPUTS_TELEM4.4
IN17
  Top 0.254: INPUTS_TELEM5.1 80.01,96.55 80.01,84.33 86.36,84.33 LMC6484_5.3
IN18
  Top 0.254: INPUTS_TELEM5.2 85.09,96.55 85.09,85.85 91.44,85.85 LMC6484_5.5
IN19
  Top 0.254: INPUTS_TELEM5.3 91.44,96.55 LMC6484_5.10
IN20
  Top 0.254: INPUTS_TELEM5.4 98.04,96.55 98.04,87.12 86.36,87.12 LMC6484_5.12
IN21
  Top 0.254: INPUTS_TELEM6.1 56.9,96.55 56.9,83.82 63.5,83.82 LMC6484_6.3
IN22
  Top 0.254: INPUTS_TELEM6.2 62.23,96.55 62.23,85.85 68.58,85.85 LMC6484_6.5
IN23
  Top 0.254: INPUTS_TELEM6.3 68.58,96.55 LMC6484_6.10
IN24
  Top 0.254: INPUTS_TELEM6.4 76.45,96.55 76.45,87.38 63.5,87.38 LMC6484_6.12
IN25
  Top 0.254: INPUTS_MOTOR1.1 33.78,96.55 33.78,84.07 40.64,84.07 LMC6484_7.3
IN26
  Top 0.254: INPUTS_MOTOR1.2 39.37,96.55 39.37,85.85 45.72,85.85 LMC6484_7.5
IN27
  Top 0.254: INPUTS_MOTOR1.3 45.72,96.55 LMC6484_7.10
IN28
  Top 0.254: INPUTS_MOTOR1.4 52.32,96.55 52.32,87.63 40.64,87.63 LMC6484_7.12
IN29
  Top 0.254: INPUTS_MOTOR2.1 11.18,96.55 11.18,83.82 17.78,83.82 LMC6484_8.3
IN30
  Top 0.254: INPUTS_MOTOR2.2 16.51,96.55 16.51,85.85 22.86,85.85 LMC6484_8.5
IN31
  Top 0.254: INPUTS_MOTOR2.3 22.86,96.55 LMC6484_8.10
IN32
  Top 0.254: INPUTS_MOTOR2.4 29.46,96.55 29.46,87.63 17.78,87.63 LMC6484_8.12
MOTOR_OVERRIDE
  Bottom 0.254: MOTOR_OVERRIDE.2 MOTOR_OVERRIDE.1
MOUNT
  pour Bottom: 151.13,3.81 5.33,3.81 5.33,1.27 151.13,1.27
  pour Bottom: 151.13,3.81 148.59,3.81 148.59,99.06 151.13,99.06
  pour Bottom: 1.52,101.6 1.52,1.27 5.33,1.27 5.33,101.6
  pour Bottom: 5.33,99.06 151.13,99.06 151.13,101.6 5.33,101.6
N$1
  Bottom 0.254: LM317.1 R1.2 136.91,53.85 119.13,53.85 R2.1
N$2
  Top 0.254: U$2.NO_2 162.56,15.24 170.18,22.86 171.45,22.86 U$2.NC_1
  Bottom 0.254: U$4.NO_1 162.56,36.83 162.56,30.48 170.18,22.86 171.45,22.86 U$2.NC_1
N$3
  Bottom 0.254: 780CAP1.1 IC1.3
N$4
  Top 0.254: Q1.C 200.66,25.4 204.47,25.4 205.74,24.13 205.74,15.24 | 205.74,15.24 205.74,5.08 U$3.IN | 205.74,15.24 187.96,15.24 U$2.COIL1
N$5
  Bottom 0.254: R4.2 175.26,44.45 179.07,44.45 184.15,39.37 184.15,7.62 187.96,7.62 SV1.2
N$6
  Bottom 0.254: U$5.IN 195.58,21.59 | 195.58,21.59 Q2.C | 195.58,21.59 187.96,29.21 U$4.COIL1
N$7
  Bottom 0.254: R3.1 190.5,30.48 Q1.B
N$8
  Bottom 0.254: R3.2 177.8,13.97 182.88,8.89 182.88,5.08 SV1.1
N$9
  Bottom 0.254: R4.1 163.83,45.72 179.07,45.72 185.42,39.37 185.42,16.51 Q2.B
N$10
  Top 0.254: C5.2 C6.2 | C5.2 C4.2 | C5.2 IC5.2 | IC4.2 198.12,69.85 200.66,69.85 | 203.2,69.85 200.66,69.85 | 203.2,69.85 203.2,63.5 X3.1 | 203.2,69.85 X5.2 | C2.2 C3.2 186.69,80.01 186.69,74.93 X6.2 | C1.2 187.96,83.82 C2.2 | C2.2 IC6.2 | 200.66,69.85 200.66,81.28 203.2,81.28 X4.2
  Bottom 0.254: IC5.2 198.12,63.5 203.2,63.5 X3.1 | IC6.2 200.66,83.82 203.2,81.28 X4.2
N$11
  Bottom 0.254: C2.1 185.42,85.09 201.93,85.09 | 201.93,85.09 203.2,86.36 X4.1 | IC4.3 205.74,80.01 205.74,85.09 201.93,85.09
N$12
  Top 0.254: IC5.3 193.04,55.88 185.42,55.88 185.42,64.77 C4.1
  Bottom 0.254: C4.1 187.96,68.58 196.85,68.58 203.2,74.93 X5.1
N$13
  Top 0.254: C5.1 181.61,63.5 181.61,69.85 184.15,69.85 186.69,72.39 | 186.69,69.85 X6.1 186.69,69.83 186.69,72.39 | 186.69,72.39 IC6.3
N$14
  Top 0.254: LMC6484_3.12 69.09,14.48 57.4,14.48 57.4,6.35 58.67,6.35 INPUTS_TELEM3.4
N$15
  Top 0.254: C1.1 190.5,86.36 IC6.1 198.12,83.82 198.12,74.93 IC4.1 193.04,72.39 193.04,63.5 IC5.1 198.12,63.5 203.2,58.42 X3.2
  Bottom 0.254: C3.1 189.23,74.93 IC4.1 | C6.1 186.69,59.69 191.77,59.69 IC5.1
N$16
  Bottom 0.254: R6.S 222.25,21.59 R5.A
N$17
  Bottom 0.254: R6.A 217.17,19.05 217.17,6.35 218.44,6.35 X18.3
N$18
  Bottom 0.254: R27.2 228.6,6.35 X18.1
N$19
  Bottom 0.254: R28.1 213.36,17.53 218.44,22.86 228.6,22.86 229.87,21.59 229.87,19.05 R5.S
N$20
  Bottom 0.254: R7.1 59.69,116.84 | 59.69,116.84 R8.2 | 59.69,116.84 59.69,110.49 X7.2
N$21
  Bottom 0.254: R8.1 49.53,121.92 54.61,127 64.77,127 66.04,125.73 66.04,123.19 R9.S
N$22
  Bottom 0.254: R10.S 58.42,125.73 R9.A
N$23
  Bottom 0.254: R10.A 53.34,123.19 53.34,110.49 54.61,110.49 X7.3
N$24
  Bottom 0.254: R7.2 69.85,110.49 64.77,110.49 X7.1
N$25
  Bottom 0.254: R11.1 86.36,116.84 | 86.36,116.84 R12.2 | 86.36,116.84 86.36,110.49 X8.2
N$26
  Bottom 0.254: R12.1 76.2,121.92 81.28,127 91.44,127 92.71,125.73 92.71,123.19 R13.S
N$27
  Bottom 0.254: R14.S 85.09,125.73 R13.A
N$28
  Bottom 0.254: R14.A 80.01,123.19 80.01,110.49 81.28,110.49 X8.3
N$29
  Bottom 0.254: R11.2 91.44,110.49 X8.1
N$30
  Bottom 0.254: R15.1 113.03,116.84 | 113.03,116.84 R16.2 | 113.03,116.84 113.03,110.49 X9.2
N$31
  Bottom 0.254: R16.1 102.87,121.92 107.95,127 118.11,127 119.38,125.73 119.38,123.19 R17.S
N$32
  Bottom 0.254: R18.S 111.76,125.73 R17.A
N$33
  Bottom 0.254: R18.A 106.68,123.19 106.68,110.49 107.95,110.49 X9.3
N$34
  Bottom 0.254: R15.2 121.92,115.57 118.11,110.49 X9.1
N$35
  Bottom 0.254: R19.1 86.36,143.51 | 86.36,143.51 R20.2 | 86.36,143.51 86.36,137.16 X10.2
N$36
  Bottom 0.254: R20.1 76.2,148.59 81.28,153.67 91.44,153.67 92.71,152.4 92.71,149.86 R21.S
N$37
  Bottom 0.254: R22.S 85.09,152.4 R21.A
N$38
  Bottom 0.254: R22.A 80.01,149.86 80.01,137.16 81.28,137.16 X10.3
N$39
  Bottom 0.254: R19.2 91.44,137.16 X10.1
N$40
  Bottom 0.254: R23.1 113.03,143.51 | 113.03,143.51 R24.2 | 113.03,143.51 113.03,137.16 X11.2
N$41
  Bottom 0.254: R25.S R24.1
N$42
  Bottom 0.254: R25.A 111.76,149.86 R26.S
N$43
  Bottom 0.254: R26.A 115.57,153.67 107.95,153.67 101.6,147.32 101.6,137.16 107.95,137.16 X11.3
N$44
  Bottom 0.254: R23.2 118.11,137.16 X11.1
N$45
  Bottom 0.254: R29.1 139.7,143.51 | 139.7,143.51 R30.2 | 139.7,143.51 139.7,137.16 X12.2
N$46
  Bottom 0.254: R30.1 129.54,148.59 134.62,153.67 144.78,153.67 146.05,152.4 146.05,149.86 R31.S
N$47
  Bottom 0.254: R32.S 138.43,152.4 R31.A
N$48
  Bottom 0.254: R32.A 133.35,149.86 133.35,137.16 134.62,137.16 X12.3
N$49
  Bottom 0.254: R27.1 223.52,12.7 | 223.52,12.7 R28.2 | 223.52,12.7 223.52,6.35 X18.2
N$50
  Bottom 0.254: R29.2 144.78,137.16 X12.1
N$51
  Bottom 0.254: R33.1 139.7,116.84 | 139.7,116.84 R34.2 | 139.7,116.84 139.7,110.49 X13.2
N$52
  Bottom 0.254: R34.1 129.54,121.92 134.62,127 144.78,127 146.05,125.73 146.05,123.19 R35.S
N$53
  Bottom 0.254: R36.S 138.43,125.73 R35.A
N$54
  Bottom 0.254: R36.A 133.35,123.19 133.35,110.49 134.62,110.49 X13.3
N$55
  Bottom 0.254: R33.2 144.78,110.49 X13.1
N$56
  Bottom 0.254: R37.1 193.04,107.95 | 193.04,107.95 R38.2 | 193.04,107.95 193.04,101.6 X14.2
N$57
  Bottom 0.254: R38.1 182.88,113.03 187.96,118.11 198.12,118.11 199.39,116.84 199.39,114.3 R39.S
N$58
  Bottom 0.254: R40.S 191.77,116.84 R39.A
N$59
  Bottom 0.254: R40.A 186.69,114.3 186.69,101.6 187.96,101.6 X14.3
N$60
  Bottom 0.254: R37.2 198.12,101.6 X14.1
N$61
  Bottom 0.254: R41.1 193.04,134.62 | 193.04,134.62 R42.2 | 193.04,134.62 193.04,128.27 X15.2
N$62
  Bottom 0.254: R42.1 182.88,139.7 187.96,144.78 198.12,144.78 199.39,143.51 199.39,140.97 R43.S
N$63
  Bottom 0.254: R44.S 191.77,143.51 R43.A
N$64
  Bottom 0.254: R44.A 186.69,140.97 186.69,128.27 187.96,128.27 X15.3
N$65
  Bottom 0.254: R41.2 198.12,128.27 X15.1
N$66
  Bottom 0.254: R45.1 166.37,116.84 | 166.37,116.84 R46.2 | 166.37,116.84 166.37,110.49 X16.2
N$67
  Bottom 0.254: R46.1 156.21,121.92 161.29,127 171.45,127 172.72,125.73 172.72,123.19 R47.S
N$68
  Bottom 0.254: R48.S 165.1,125.73 R47.A
N$69
  Bottom 0.254: R48.A 160.02,123.19 160.02,110.49 161.29,110.49 X16.3
N$70
  Bottom 0.254: R45.2 171.45,110.49 X16.1
N$71
  Bottom 0.254: R49.1 166.37,143.51 | 166.37,143.51 R50.2 | 166.37,143.51 166.37,137.16 X17.2
N$72
  Bottom 0.254: R50.1 156.21,148.59 161.29,153.67 171.45,153.67 172.72,152.4 172.72,149.86 R51.S
N$73
  Bottom 0.254: R52.S 165.1,152.4 R51.A
N$74
  Bottom 0.254: R52.A 160.02,149.86 160.02,137.16 161.29,137.16 X17.3
N$75
  Bottom 0.254: R49.2 171.45,137.16 X17.1
N$76
  Bottom 0.254: R53.1 223.52,119.38 | 223.52,119.38 R54.2 | 223.52,119.38 223.52,113.03 X19.2
N$77
  Bottom 0.254: R54.1 213.36,124.46 218.44,129.54 228.6,129.54 229.87,128.27 229.87,125.73 R55.S
N$78
  Bottom 0.254: R56.S 222.25,128.27 R55.A
N$79
  Bottom 0.254: R56.A 217.17,125.73 217.17,113.03 218.44,113.03 X19.3
N$80
  Bottom 0.254: R53.2 228.6,113.03 X19.1
N$81
  Bottom 0.254: R57.1 166.37,90.17 | 166.37,90.17 R58.2 | 166.37,90.17 166.37,83.82 X20.2
N$82
  Bottom 0.254: R58.1 156.21,95.25 161.29,100.33 171.45,100.33 172.72,99.06 172.72,96.52 R59.S
N$83
  Bottom 0.254: R60.S 165.1,99.06 R59.A
N$84
  Bottom 0.254: R60.A 160.02,96.52 160.02,83.82 161.29,83.82 X20.3
N$85
  Bottom 0.254: R57.2 171.45,83.82 X20.1
N$86
  Bottom 0.254: R61.1 166.37,63.5 | 166.37,63.5 R62.2 | 166.37,63.5 166.37,57.15 X21.2
N$87
  Bottom 0.254: R62.1 156.21,68.58 161.29,73.66 171.45,73.66 172.72,72.39 172.72,69.85 R63.S
N$88
  Bottom 0.254: R64.S 165.1,72.39 R63.A
N$89
  Bottom 0.254: R64.A 160.02,69.85 160.02,57.15 161.29,57.15 X21.3
N$90
  Bottom 0.254: R61.2 171.45,57.15 X21.1
N$91
  Bottom 0.254: R65.1 223.52,92.71 | 223.52,92.71 R66.2 | 223.52,92.71 223.52,86.36 X22.2
N$92
  Bottom 0.254: R66.1 213.36,97.79 218.44,102.87 228.6,102.87 229.87,101.6 229.87,99.06 R67.S
N$93
  Bottom 0.254: R68.S 222.25,101.6 R67.A
N$94
  Bottom 0.254: R68.A 217.17,99.06 217.17,86.36 218.44,86.36 X22.3
N$95
  Bottom 0.254: R65.2 228.6,86.36 X22.1
N$96
  Bottom 0.254: R69.1 223.52,39.37 | 223.52,39.37 R70.2 | 223.52,39.37 223.52,33.02 X23.2
N$97
  Bottom 0.254: R70.1 213.36,44.45 218.44,49.53 228.6,49.53 229.87,48.26 229.87,45.72 R71.S
N$98
  Bottom 0.254: R72.S 222.25,48.26 R71.A
N$99
  Bottom 0.254: R72.A 217.17,45.72 217.17,33.02 218.44,33.02 X23.3
N$100
  Bottom 0.254: R69.2 228.6,33.02 X23.1
N$101
  Bottom 0.254: R73.1 223.52,66.04 | 223.52,66.04 R74.2 | 223.52,66.04 223.52,59.69 X24.2
N$102
  Bottom 0.254: R74.1 213.36,71.12 218.44,76.2 228.6,76.2 229.87,74.93 229.87,72.39 R75.S
N$103
  Bottom 0.254: R76.S 222.25,74.93 R75.A
N$104
  Bottom 0.254: R76.A 217.17,72.39 217.17,59.69 218.44,59.69 X24.3
N$105
  Bottom 0.254: R73.2 228.6,59.69 X24.1
N$106
  Bottom 0.254: INTERNAL_TEMP_SENSOR1.V+ 226.06,139.7 228.6,139.7 X25.1
N$107
  Bottom 0.254: INTERNAL_TEMP_SENSOR1.VOUT 220.98,139.7 223.52,139.7 X25.2
N$108
  Bottom 0.254: INTERNAL_TEMP_SENSOR1.GND 220.98,149.86 218.44,147.32 218.44,139.7 X25.3
N$109
  Bottom 0.254: INTERNAL_TEMP_SENSOR2.V+ 11.43,138.43 6.35,138.43 X26.1
N$110
  Bottom 0.254: INTERNAL_TEMP_SENSOR2.VOUT 11.43,143.51 6.35,143.51 X26.2
N$111
  Bottom 0.254: INTERNAL_TEMP_SENSOR2.GND 16.51,146.05 16.51,148.59 6.35,148.59 X26.3
N$112
  Bottom 0.254: INTERNAL_TEMP_SENSOR3.V+ 11.43,111.76 6.35,111.76 X27.1
N$113
  Bottom 0.254: INTERNAL_TEMP_SENSOR3.VOUT 11.43,116.84 6.35,116.84 X27.2
N$114
  Bottom 0.254: INTERNAL_TEMP_SENSOR3.GND 16.51,119.38 16.51,121.92 6.35,121.92 X27.3
N$115
  Bottom 0.254: INTERNAL_TEMP_SENSOR4.V+ 198.12,153.67 X28.1
N$116
  Bottom 0.254: INTERNAL_TEMP_SENSOR4.VOUT 185.67,156.21 185.67,151.13 190.5,151.13 193.04,153.67 X28.2
N$117
  Bottom 0.254: INTERNAL_TEMP_SENSOR4.GND 187.96,156.21 187.96,153.67 X28.3
N$118
  Bottom 0.254: INTERNAL_TEMP_SENSOR5.V+ 62.23,137.16 64.77,137.16 X29.1
N$119
  Bottom 0.254: INTERNAL_TEMP_SENSOR5.VOUT 57.15,137.16 59.69,137.16 X29.2
N$120
  Bottom 0.254: INTERNAL_TEMP_SENSOR5.GND 57.15,147.32 54.61,144.78 54.61,137.16 X29.3
N$121
  Bottom 0.254: INTERNAL_TEMP_SENSOR6.V+ 35.56,129.54 38.1,129.54 X30.1
N$122
  Bottom 0.254: INTERNAL_TEMP_SENSOR6.VOUT 30.48,129.54 33.02,129.54 X30.2
N$123
  Bottom 0.254: INTERNAL_TEMP_SENSOR6.GND 30.48,139.7 27.94,137.16 27.94,129.54 X30.3
N$124
  Bottom 0.254: INTERNAL_TEMP_SENSOR7.V+ 35.56,110.49 38.1,110.49 X31.1
N$125
  Bottom 0.254: INTERNAL_TEMP_SENSOR7.VOUT 30.48,110.49 33.02,110.49 X31.2
N$126
  Bottom 0.254: INTERNAL_TEMP_SENSOR7.GND 30.48,120.65 27.94,118.11 27.94,110.49 X31.3
N$127
  Bottom 0.254: INTERNAL_TEMP_SENSOR8.V+ 34.29,148.59 36.83,148.59 X32.1
N$128
  Bottom 0.254: INTERNAL_TEMP_SENSOR8.VOUT 29.21,148.59 31.75,148.59 X32.2
N$129
  Bottom 0.254: INTERNAL_TEMP_SENSOR8.GND 29.21,158.75 26.67,156.21 26.67,148.59 X32.3
PURPLE
  Top 0.254: U$2.COM_1 167.64,15.24 175.26,7.62 175.26,6.35 X2.2
SPI_CLK  (via drill 0.8)
  Top 0.254: v75.18,49.53 91.69,49.53 114.3,26.67 130.84,26.67 SPI_TELEM.1 | v50.04,43.69 50.04,44.96 66.29,44.96 69.34,41.91 74.93,41.91 U$14.13
  Bottom 0.254: U$16.13 77.98,53.59 v75.18,49.53 75.18,40.64 U$14.13 | U$1.13 27.69,43.69 v50.04,43.69
SPI_CLK_MOTOR
  Top 0.254: SPI_MOTOR.1 142.22,77.49 132.08,86.36 115.57,86.36 90.42,54.61 33.27,54.61 U$17.13
SPI_CS1
  Top 0.254: U$1.10 35.81,41.66 35.81,45.72 87.88,45.72 110.49,22.86 142.26,22.86 SPI_TELEM.4
SPI_CS2  (via drill 0.8)
  Top 0.254: v84.07,44.45 87.88,44.45 109.22,21.59 SPI_TELEM.5
  Bottom 0.254: U$14.10 83.57,43.94 v84.07,44.45
SPI_CS3  (via drill 0.8)
  Top 0.254: v70.1,43.18 86.61,43.18 107.95,20.32 142.24,20.32 146.05,16.51 SPI_TELEM.6
  Bottom 0.254: U$16.10 70.36,43.43 v70.1,43.18
SPI_CS4
  Top 0.254: SPI_MOTOR.4 146.07,63.48 142.24,67.31 128.27,82.55 119.38,82.55 95.5,50.8 25.65,50.8 U$17.10
SPI_DIN  (via drill 0.8)
  Top 0.254: U$1.11 33.27,41.4 33.27,46.99 v71.37,46.99 v81.53,46.99 89.15,46.99 111.76,24.13 138.46,24.13 SPI_TELEM.3
  Bottom 0.254: v81.53,46.99 81.53,41.4 U$14.11 | U$16.11 72.9,51.05 71.37,49.53 v71.37,46.99
SPI_DIN_MOTOR
  Top 0.254: SPI_MOTOR.3 146.07,68.56 129.54,83.82 118.11,83.82 92.96,52.07 28.19,52.07 U$17.11
SPI_DOUT  (via drill 0.8)
  Top 0.254: U$1.12 30.73,41.4 30.73,48.26 v73.15,48.26 v77.72,48.26 90.42,48.26 113.03,25.4 134.62,25.4 146.05,36.83 SPI_TELEM.2
  Bottom 0.254: v77.72,48.26 77.72,41.66 U$14.12 | U$16.12 75.44,52.32 73.15,49.53 v73.15,48.26
SPI_DOUT_MOTOR
  Top 0.254: SPI_MOTOR.2 144.76,72.41 130.81,85.09 116.84,85.09 91.69,53.34 30.73,53.34 U$17.12
VREF  (via drill 0.61, 0.8)
  Top 0.254: v106.68,63.5 114.3,55.88 IC1.6 | U$14.15 70.87,37.34 71.37,36.83 v86.61,36.83 | v37.08,55.88 37.08,60.96 U$17.15
  Bottom 0.254: IC1.6 780CAP2.1 | U$17.15 39.62,63.5 81.53,63.5 U$16.15 84.07,60.96 92.96,60.96 | v106.68,63.5 104.14,60.96 92.96,60.96 | v86.61,36.83 87.88,36.83 92.96,41.91 92.96,60.96 | U$1.15 22.61,41.4 v37.08,55.88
